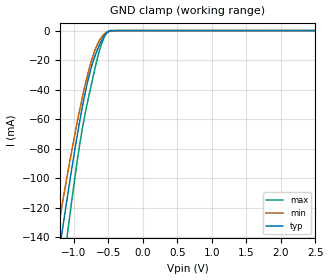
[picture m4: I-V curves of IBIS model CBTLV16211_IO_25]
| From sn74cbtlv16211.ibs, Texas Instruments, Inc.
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[Model]   CBTLV16211_IO_25
Model_type  Terminator
| variable   typ   min   max
C_comp   4.02pF   3.46pF   4.47pF
| C_tri-state   4.02pF   3.46pF   4.47pF
[Temperature Range]   40   100   -40
| Ambient temperature   25   85   -40
[Voltage range]   2.5   2.3   2.7
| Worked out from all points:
|   GND clamp passes 1 mA (typ) near -0.52 V on its own axis
[GND Clamp]
| CBTLV16211_IO_25
|   Voltage   I(typ)   I(min)   I(max)
-5.5V     -1.743A    -1.502A    -2.1A
-1.26V    -165mA     -142.4mA   -201.6mA
-1.22V    -152mA     -131.3mA   -185.9mA
-1.185V   -140.8mA   -121.8mA   -172.3mA
-1.15V    -129.8mA   -112.3mA   -158.9mA
-1.115V   -118.8mA   -103mA     -145.7mA
-1.085V   -109.6mA   -95.11mA   -134.6mA
-920mV    -62.43mA   -54.52mA   -78.32mA
-795mV    -33.36mA   -28.61mA   -46.68mA
-630mV    -9.728mA   -6.608mA   -13.42mA
-500mV    -466.3uA   -767.1uA   -499.5uA
2.5V      1.214nA    60.76nA    11.78pA
